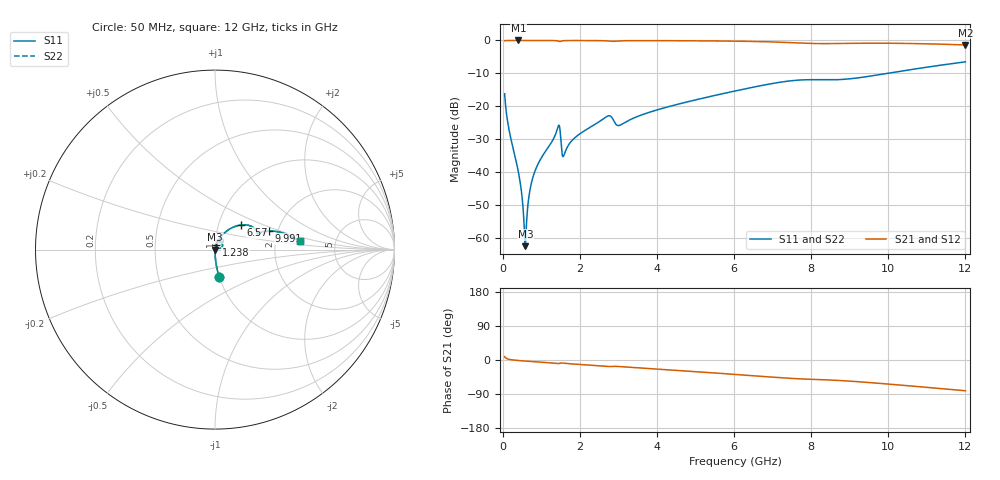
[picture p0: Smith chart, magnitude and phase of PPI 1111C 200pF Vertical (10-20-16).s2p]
# GHz S MA R 50
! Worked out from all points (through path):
!   1601 points, 50 MHz to 12 GHz, reference 50 ohm
!   highest |S21| = -0.01 dB at 408.5 MHz (marker M1); lowest = -1.4 dB at 12 GHz (marker M2)
!   group delay of S21, straight-line fit = 18.5 ps
!   lowest |S11| = -62.3 dB at 587.8 MHz (marker M3), VSWR 1.00, Z = 50.1 + j0.00997 ohm
!   |S11| at or under -10 dB: start of sweep to 9.965 GHz
!   |S22| runs from -62.3 to -6.5 dB; largest |S21 - S12| = 0
!   S11 on the Smith chart (normalised r, x): 50 MHz: 1.00, -0.32; 1.238 GHz: 1.01, +0.05; 6.57 GHz: 1.28, +0.37; 9.991 GHz: 1.80, +0.42; 12 GHz: 2.75, +0.33
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0.05  0.1557 -81.2  0.9875 8.7  0.9875 8.7  0.1557 -81.2
0.1769688  0.04079 -87.9  0.9987 1.5  0.9987 1.5  0.04079 -87.9
0.4085  0.01006 -87.7  0.9993 -1.4  0.9993 -1.4  0.01006 -87.7
0.4831875  0.005328 -84.6  0.9993 -2.0  0.9993 -2.0  0.005328 -84.6
0.5504062  0.00183 -69.0  0.9992 -2.5  0.9992 -2.5  0.00183 -69.0
0.58775  0.0007649 7.5  0.9992 -2.8  0.9992 -2.8  0.0007649 7.5
0.6250938  0.002006 64.2  0.9992 -3.1  0.9992 -3.1  0.002006 64.2
0.70725  0.005416 77.5  0.9991 -3.7  0.9991 -3.7  0.005416 77.5
0.796875  0.008939 80.0  0.999 -4.3  0.999 -4.3  0.008939 80.0
1.237531  0.02695 78.5  0.9977 -7.5  0.9977 -7.5  0.02695 78.5
1.439188  0.04988 56.0  0.9782 -9.5  0.9782 -9.5  0.04988 56.0
1.596031  0.01873 59.0  0.9926 -8.6  0.9926 -8.6  0.01873 59.0
2.044156  0.04004 74.8  0.9969 -12.1  0.9969 -12.1  0.04004 74.8
2.723813  0.07145 59.6  0.9809 -17.0  0.9809 -17.0  0.07145 59.6
3.022562  0.05154 56.4  0.9841 -17.2  0.9841 -17.2  0.05154 56.4
4.038312  0.08986 63.5  0.9922 -24.3  0.9922 -24.3  0.08986 63.5
6.025  0.1714 48.9  0.9758 -38.0  0.9758 -38.0  0.1714 48.9
6.570219  0.1997 43.4  0.9638 -42.1  0.9638 -42.1  0.1997 43.4
8.019156  0.2544 23.1  0.8998 -51.0  0.8998 -51.0  0.2544 23.1
9.990906  0.318 19.1  0.9071 -63.4  0.9071 -63.4  0.318 19.1
10.01331  0.3196 19.0  0.9069 -63.6  0.9069 -63.6  0.3196 19.0
12  0.4737 5.7  0.8546 -81.2  0.8546 -81.2  0.4737 5.7
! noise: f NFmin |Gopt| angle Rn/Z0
0.05  0.0003684  0.8648  0.3357  0.0005851
1.372  0.008662  0.8444  6.546  0.01178
2.701  0.01891  0.8595  12.84  0.02846
4.031  0.01151  0.6909  18.75  0.007064
5.36  0.01652  0.7145  24.72  0.01092
6.682  0.03319  0.8162  30.83  0.03512
8.012  0.07254  0.8972  36.75  0.1388
9.341  0.06808  0.877  42.26  0.1041
10.67  0.05677  0.8399  47.41  0.06305
12  0.05354  0.8176  52.28  0.04964
